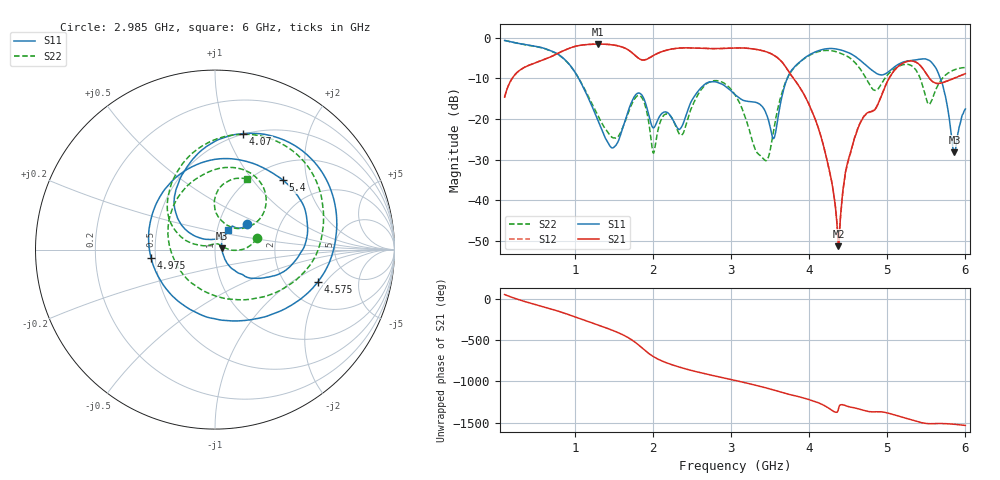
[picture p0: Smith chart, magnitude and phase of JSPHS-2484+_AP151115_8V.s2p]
!Mini-Circuits Laboratory
!S-Parameters
!Run/Lot/Date Code:MF33450/NA/1551
!Fixture/SN/Due: 90-4-20-21/70546/03/17/16
!Connection:PORT<IN> - pin<1>; PORT<OUT> - pin<7>;PORT<BIAS> - pin<4>;
!Tested With:PORT EXTENTION
!Network Analyzer:AG E5071C/74883/05/12/16
!Created: 01-07-2016 at 14:10:14
!MODEL: JSPHS-2484+
!S/N: V=8V
# MHZ S DB R 50
!Frequency  S11 dB  S11 DEG  S21 dB  S21 DEG  S12 dB  S12 DEG  S22 dB  S22 DEG
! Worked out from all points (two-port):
!   1181 points, 100 MHz to 6 GHz, reference 50 ohm
!   highest |S21| = -1.55 dB at 1.3 GHz (marker M1); lowest = -51.3 dB at 4.375 GHz (marker M2)
!   |S21| within 3 dB of the highest: 706.9 MHz to 1.784 GHz (1.077 GHz wide, 86.5 % of centre); 1.988 GHz to 3.568 GHz (1.58 GHz wide, 56.9 % of centre)
!   lowest |S11| = -28.1 dB at 5.86 GHz (marker M3), VSWR 1.08, Z = 54 + j0.867 ohm
!   |S11| at or under -10 dB: 1.048 GHz to 3.719 GHz (2.671 GHz wide, 112 % of centre); 5.68 GHz to end of sweep
!   |S22| runs from -30.2 to -0.7 dB; largest |S21 - S12| = 0.0024
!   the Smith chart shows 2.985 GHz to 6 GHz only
!   S11 on the Smith chart (normalised r, x): 2.985 GHz: 1.37, +0.41; 4.07 GHz: 0.49, +1.14; 4.575 GHz: 3.00, -1.67; 4.975 GHz: 0.47, -0.05; 5.4 GHz: 1.32, +1.45; 6 GHz: 1.13, +0.25
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100  -0.67 -40.0  -14.61 49.7  -14.60 49.7  -0.66 -39.9
515  -2.17 -165.1  -6.00 -77.0  -6.00 -77.0  -2.21 -168.3
800  -4.25 118.8  -3.66 -155.4  -3.66 -155.5  -4.32 114.6
1085  -11.33 26.8  -1.80 111.2  -1.80 111.2  -11.20 22.4
1300  -20.56 -47.1  -1.55 39.7  -1.55 39.7  -19.37 -60.0
1600  -22.93 167.5  -2.24 -71.0  -2.23 -71.0  -22.66 -171.4
1775  -14.10 83.5  -4.41 -170.4  -4.41 -170.4  -14.74 98.7
1910  -16.43 19.6  -5.36 83.3  -5.36 83.2  -17.36 16.5
2070  -19.84 48.4  -3.74 -14.5  -3.74 -14.5  -22.22 68.5
2550  -13.84 80.7  -2.54 -162.5  -2.53 -162.5  -14.89 83.3
2985  -12.80 38.1  -2.55 104.7  -2.55 104.7  -12.39 15.2
3050  -13.99 38.4  -2.50 91.0  -2.50 90.9  -14.04 6.8
3450  -18.68 52.2  -3.44 -0.3  -3.44 -0.4  -30.22 100.4
4035  -3.85 82.1  -18.00 -152.1  -18.01 -152.0  -4.02 85.7
4070  -3.55 76.4  -19.67 -163.0  -19.66 -162.8  -3.73 79.7
4375  -2.87 22.9  -51.27 104.4  -49.61 102.4  -3.63 25.4
4575  -4.42 -17.2  -25.05 119.5  -24.95 120.8  -5.89 -15.0
4975  -8.88 -172.9  -11.85 62.8  -11.85 62.6  -9.83 139.0
5020  -8.29 162.5  -10.06 52.6  -10.08 52.4  -8.77 122.2
5400  -5.32 45.5  -6.42 -51.1  -6.42 -51.2  -9.05 38.5
5860  -28.15 11.8  -9.94 -80.0  -9.93 -80.0  -7.88 76.0
6000  -17.52 56.0  -8.83 -94.4  -8.82 -94.4  -7.32 65.8
